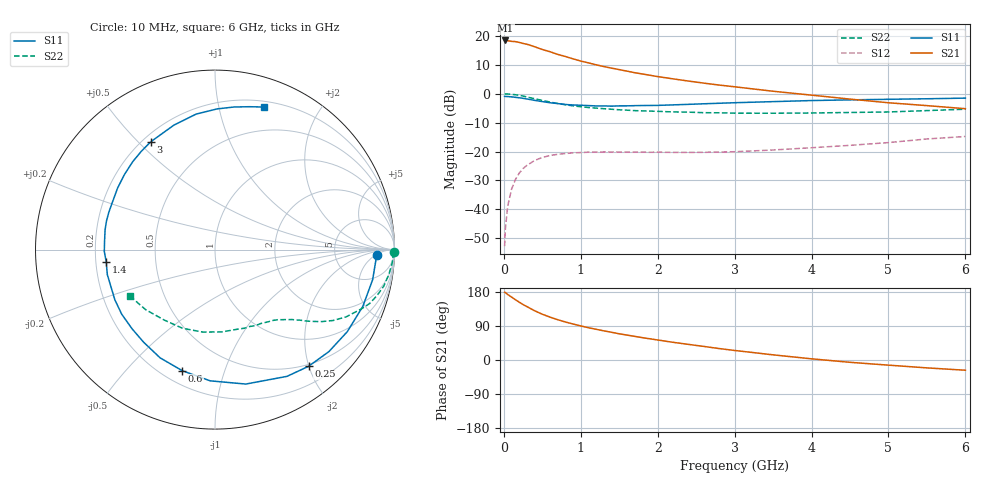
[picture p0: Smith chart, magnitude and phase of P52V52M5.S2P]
! SIEMENS Small Signal Semiconductors
! BFP183
! Si NPN RF Bipolar Junction Transistor in SOT143
! VCE = 2.5 V  IC = 2.5 mA
! Common Emitter S-Parameters:  March  1996
# GHz  S  MA  R  50
!  f  S11  S21  S12  S22
! GHz  MAG  ANG  MAG  ANG  MAG  ANG  MAG  ANG
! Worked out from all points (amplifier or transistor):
!   36 points, 10 MHz to 6 GHz, reference 50 ohm
!   highest |S21| = 18.4 dB at 20 MHz (marker M1)
!   |S21| within 3 dB of that: start of sweep to 486.5 MHz
!   unconditionally stable (mu >= 1): 1.958 GHz to 5.777 GHz
!   at 250 MHz: K = 0.14, MSG = 21.6 dB, |S12| = -25.9 dB
!   at 1.4 GHz: K = 0.74, MSG = 14.5 dB, |S12| = -20.2 dB
!   at 6 GHz: K = 0.96, MSG = 4.8 dB, |S12| = -14.8 dB
!   S11 on the Smith chart (normalised r, x): 10 MHz: 17, -6; 250 MHz: 0.47, -1.99; 600 MHz: 0.28, -0.73; 1.4 GHz: 0.24, -0.05; 3 GHz: 0.23, +0.54; 6 GHz: 0.25, +1.37
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0.01  0.9009 -2.0  8.252 178.9  0.0023 85.8  0.9973 -0.9
0.02  0.8975 -4.3  8.364 177.8  0.0046 89.6  0.9926 -1.7
0.05  0.8942 -10.8  8.275 173.0  0.0113 87.6  0.9903 -4.2
0.15  0.8674 -31.8  7.997 159.1  0.0327 72.1  0.9616 -12.3
0.2  0.852 -41.8  7.741 152.6  0.0423 67.6  0.9379 -15.9
0.25  0.8334 -51.3  7.413 146.3  0.0507 62.1  0.9118 -19.3
0.3  0.8122 -60.4  7.198 140.9  0.0577 57.9  0.8793 -22.1
0.4  0.7685 -77.1  6.512 129.9  0.0699 49.6  0.8206 -27.2
0.5  0.7317 -92.1  5.834 120.8  0.0789 42.8  0.767 -31.0
0.6  0.699 -105.1  5.336 113.2  0.0854 37.4  0.7189 -33.9
0.7  0.6762 -116.9  4.802 106.4  0.0895 33.0  0.6779 -36.2
0.8  0.6515 -127.6  4.41 100.3  0.0923 29.3  0.6449 -38.1
0.9  0.6389 -136.3  4.018 95.0  0.0948 26.5  0.6169 -39.6
1.1  0.6241 -153.4  3.423 85.1  0.0974 21.9  0.5776 -42.4
1.4  0.6099 -173.5  2.777 73.2  0.0982 17.3  0.5393 -46.4
1.8  0.6252 165.2  2.2 59.0  0.0975 15.2  0.5055 -51.7
2.2  0.6418 147.8  1.811 46.7  0.0966 15.0  0.4845 -58.2
3  0.6993 120.8  1.32 25.2  0.0992 18.8  0.4611 -73.9
3.5  0.7306 108.2  1.105 13.6  0.1063 21.8  0.4602 -85.0
4.5  0.7837 89.2  0.808 -6.1  0.1279 24.4  0.4741 -112.4
5.5  0.8187 76.5  0.623 -20.8  0.1649 23.0  0.5109 -139.0
6  0.8402 71.0  0.551 -27.0  0.1821 19.6  0.5402 -151.4
